PROGRAM MAIN
VAR
	nEl1262Ch1Bits			: ARRAY[1..1000] OF BOOL;
	nEl1262Ch2Bits			: ARRAY[1..1000] OF BOOL;
	
	fbSentDecodeCh1			: FB_SENT_Decoder;
	fbSentDecodeCh2			: FB_SENT_Decoder;
	
	stSlowDatasCh1			: ARRAY[1..16] OF ST_SentSlowChnData;	// Slow-Channel-Daten des AFA 11.00 D7 Z16E L ST B632 Pressure Transmitte
	stSlowDatasCh2			: ARRAY[1..16] OF ST_SentSlowChnData;	// Slow-Channel-Daten des AFA 11.00 D7 Z16E L ST B632 Pressure Transmitte
	
	fSlowDataTemperatureCh1	: REAL;									// Temperatur die im Slow-Channel übertragen wird [°C]
	fFastDataPresureCh1		: REAL;									// Druck der im Fast-Channel übertragen wird [Pa]
	
	fSlowDataTemperatureCh2	: REAL;									// Temperatur die im Slow-Channel übertragen wird [°C]
	fFastDataPresureCh2		: REAL;									// Druck der im Fast-Channel übertragen wird [Pa]
	
	bToggle					: BOOL;
	
	nCalcCrc4				: BYTE;
	nCalcCrc4Legacy			: BYTE;
	nCalcCrc6				: BYTE;
	nCrc					: BYTE;
END_VAR

// Oversampling Daten der EL1262 von einem Byte-Array in ein Bool-Array convertieren
F_ConvByteArrToBitArr(nSrcBytes:= GVL_IO.nEl1262Ch1, nDestBits:= nEl1262Ch1Bits);
F_ConvByteArrToBitArr(nSrcBytes:= GVL_IO.nEl1262Ch2, nDestBits:= nEl1262Ch2Bits);

// Decoder aufrufen
fbSentDecodeCh1(
	bEnable:= TRUE, 
	nNominalTickTimeUs:= 10, 
	eFastChannelConfig:= E_SentFastChnConfig.eValue_MsgCnt_InvMSB, 
	eSlowChannelConfig:= E_SentSlowChnConfig.eEnhancedSerial, 
	bNewFrameStart=> , 
	nFrameLenUs=> ,  
	bNewFastChnData=> , 
	bFastChnDataValid=> , 
	nFastChnDataCnt=> , 
	bNewSlowChnData=> , 
	bSlowChnDataValid=> , 
	stRawNibbleData=> , 
	stFastChnData=> , 
	stSlowChnData=> ,
	stRxStats=>,
	nInputData:= nEl1262Ch1Bits);
	
// analyse fast-channel data of AFA 11.00 D7 Z16E L ST B632 Pressure Transmitte
IF (TO_REAL(stSlowDatasCh1[9].nData) - TO_REAL(stSlowDatasCh1[8].nData)) <> 0.0 THEN
	fFastDataPresureCh1 := TO_REAL(stSlowDatasCh1[6].nData) + (TO_REAL(stSlowDatasCh1[7].nData) - TO_REAL(stSlowDatasCh1[6].nData)) / (TO_REAL(stSlowDatasCh1[9].nData) - TO_REAL(stSlowDatasCh1[8].nData)) * (TO_REAL(fbSentDecodeCh1.stFastChnData.nValue1) - TO_REAL(stSlowDatasCh1[8].nData));
END_IF
//fFastDataPresureCh1 := 600.0 + ((120.0E4 - 600.0)/(4000.0 - 2.0)) * (TO_REAL(fbSentDecodeCh1.stFastChnData.nValue1) - 2.0);
	
// analyse slow-channel data of AFA 11.00 D7 Z16E L ST B632 Pressure Transmitte
IF fbSentDecodeCh1.bNewSlowChnData AND fbSentDecodeCh1.bSlowChnDataValid THEN
	CASE fbSentDecodeCh1.stSlowChnData.nMsgId OF
		16#1: stSlowDatasCh1[1] := fbSentDecodeCh1.stSlowChnData;
		16#3: stSlowDatasCh1[2] := fbSentDecodeCh1.stSlowChnData;
		16#4: stSlowDatasCh1[3] := fbSentDecodeCh1.stSlowChnData;
		16#5: stSlowDatasCh1[4] := fbSentDecodeCh1.stSlowChnData;
		16#6: stSlowDatasCh1[5] := fbSentDecodeCh1.stSlowChnData;
		16#7: stSlowDatasCh1[6] := fbSentDecodeCh1.stSlowChnData;
		16#8: stSlowDatasCh1[7] := fbSentDecodeCh1.stSlowChnData;
		16#9: stSlowDatasCh1[8] := fbSentDecodeCh1.stSlowChnData;
		16#A: stSlowDatasCh1[9] := fbSentDecodeCh1.stSlowChnData;
		16#10: stSlowDatasCh1[10] := fbSentDecodeCh1.stSlowChnData;
		16#12: stSlowDatasCh1[11] := fbSentDecodeCh1.stSlowChnData;
		16#13: stSlowDatasCh1[12] := fbSentDecodeCh1.stSlowChnData;
		16#14: stSlowDatasCh1[13] := fbSentDecodeCh1.stSlowChnData;
		16#15: stSlowDatasCh1[14] := fbSentDecodeCh1.stSlowChnData;
		16#29: stSlowDatasCh1[15] := fbSentDecodeCh1.stSlowChnData;
		16#2C: stSlowDatasCh1[16] := fbSentDecodeCh1.stSlowChnData;
	END_CASE
	
	
	// calc temp
	IF (TO_REAL(stSlowDatasCh1[14].nData)-TO_REAL(stSlowDatasCh1[13].nData)) <> 0.0 THEN
		fSlowDataTemperatureCh1 := (TO_REAL(stSlowDatasCh1[11].nData) + (TO_REAL(stSlowDatasCh1[12].nData)-TO_REAL(stSlowDatasCh1[11].nData))/(TO_REAL(stSlowDatasCh1[14].nData)-TO_REAL(stSlowDatasCh1[13].nData))*(TO_REAL(stSlowDatasCh1[10].nData)-TO_REAL(stSlowDatasCh1[13].nData))) / 8 - 73.15;
	END_IF
END_IF


fbSentDecodeCh2(
	bEnable:= TRUE, 
	nNominalTickTimeUs:= 3, 
	eFastChannelConfig:= E_SentFastChnConfig.eValue_MsgCnt_InvMSB, 
	eSlowChannelConfig:= E_SentSlowChnConfig.eEnhancedSerial, 
	bNewFrameStart=> , 
	nFrameLenUs=> , 
	bNewFastChnData=> , 
	bFastChnDataValid=> , 
	nFastChnDataCnt=> , 
	bNewSlowChnData=> , 
	bSlowChnDataValid=> ,
	stRawNibbleData=> , 
	stFastChnData=> , 
	stSlowChnData=> ,
	stRxStats=> ,
	nInputData:= nEl1262Ch2Bits);

// analyse fast-channel data of AFA 11.00 D7 Z16E L ST B632 Pressure Transmitte
//IF (TO_REAL(stSlowDatasCh2[9].nData) - TO_REAL(stSlowDatasCh2[8].nData)) <> 0.0 THEN
//	fFastDataPresureCh2 := TO_REAL(stSlowDatasCh2[6].nData) + (TO_REAL(stSlowDatasCh2[7].nData) - TO_REAL(stSlowDatasCh2[6].nData)) / (TO_REAL(stSlowDatasCh2[9].nData) - TO_REAL(stSlowDatasCh2[8].nData)) * (TO_REAL(fbSentDecodeCh2.stFastChnData.nValue1) - TO_REAL(stSlowDatasCh2[8].nData));
//END_IF
fFastDataPresureCh2 := 0.5 + ((13.0 - 0.5)/(to_real(16#F3D) - to_real(16#97))) * (TO_REAL(fbSentDecodeCh2.stFastChnData.nValue1) - to_real(16#97));	
	
	
// analyse slow-channel data of AFA 11.00 D7 Z16E L ST B632 Pressure Transmitte
IF fbSentDecodeCh2.bNewSlowChnData AND fbSentDecodeCh2.bSlowChnDataValid THEN
	CASE fbSentDecodeCh2.stSlowChnData.nMsgId OF
		16#1: stSlowDatasCh2[1] := fbSentDecodeCh2.stSlowChnData;
		16#3: stSlowDatasCh2[2] := fbSentDecodeCh2.stSlowChnData;
		16#4: stSlowDatasCh2[3] := fbSentDecodeCh2.stSlowChnData;
		16#80: stSlowDatasCh2[4] := fbSentDecodeCh2.stSlowChnData;
		16#6: stSlowDatasCh2[5] := fbSentDecodeCh2.stSlowChnData;
		16#7: stSlowDatasCh2[6] := fbSentDecodeCh2.stSlowChnData;
		16#8: stSlowDatasCh2[7] := fbSentDecodeCh2.stSlowChnData;
		16#9: stSlowDatasCh2[8] := fbSentDecodeCh2.stSlowChnData;
		16#A: stSlowDatasCh2[9] := fbSentDecodeCh2.stSlowChnData;
		16#10: stSlowDatasCh2[10] := fbSentDecodeCh2.stSlowChnData;
		16#12: stSlowDatasCh2[11] := fbSentDecodeCh2.stSlowChnData;
		16#13: stSlowDatasCh2[12] := fbSentDecodeCh2.stSlowChnData;
		16#14: stSlowDatasCh2[13] := fbSentDecodeCh2.stSlowChnData;
		16#15: stSlowDatasCh2[14] := fbSentDecodeCh2.stSlowChnData;
		16#29: stSlowDatasCh2[15] := fbSentDecodeCh2.stSlowChnData;
		16#2A: stSlowDatasCh2[16] := fbSentDecodeCh2.stSlowChnData;
	END_CASE
	
	
	// calc temp
	IF (TO_REAL(stSlowDatasCh2[14].nData)-TO_REAL(stSlowDatasCh2[13].nData)) <> 0.0 THEN
		fSlowDataTemperatureCh2 := (TO_REAL(stSlowDatasCh2[11].nData) + (TO_REAL(stSlowDatasCh2[12].nData)-TO_REAL(stSlowDatasCh2[11].nData))/(TO_REAL(stSlowDatasCh2[14].nData)-TO_REAL(stSlowDatasCh2[13].nData))*(TO_REAL(stSlowDatasCh2[10].nData)-TO_REAL(stSlowDatasCh2[13].nData))) / 8 - 73.15;
	END_IF
END_IF

bToggle := NOT bToggle;

END_PROGRAM
